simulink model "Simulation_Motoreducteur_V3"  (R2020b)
settings: Solver=FixedStepAuto  StartTime=0.0  StopTime=3  FixedStep=0.001  RelTol=1e-3
libraries: simulink x2

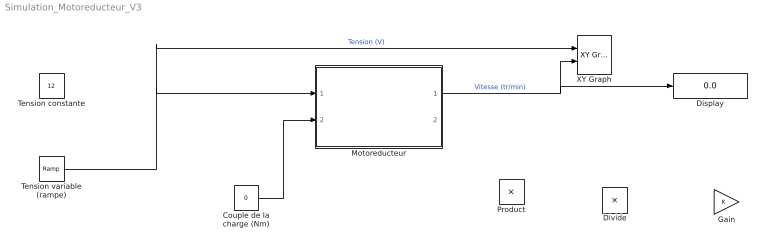
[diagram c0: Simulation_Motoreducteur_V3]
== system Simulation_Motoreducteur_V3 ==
  Couple de la charge (Nm) : Constant  Value=0
  Display : Display
  Divide : Product  Inputs=*/
  Gain : Gain
  Motoreducteur : Subsystem  mask{k=1, R=0, Io=0, r1=1, Rend=100}
      mask prompts: k "Constante de couple (Nm/A)"; R "Resistance d'induit (ohm)"; Io "Courant a vide (A)"; r1 "Rapport de reduction"; Rend "Rendement du reducteur (%)"
  Product : Product
  Tension constante : Constant  Value=12
  Tension variable (rampe) : simulink/Sources/Ramp  slope=12/3  start=0  InitialOutput=0
  XY Graph : simulink/Sinks/XY Graph  xmin=0  xmax=12  ymin=0  ymax=250  st=-1
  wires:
  Tension variable (rampe)/1 -> XY Graph/1, Motoreducteur/1(In1)  "Tension (V)"
  Motoreducteur/1(Out2) -> XY Graph/2, Display/1  "Vitesse (tr/min)"
  Motoreducteur/2(Out3) -> ?  "Courant (A)"
  Couple de la charge (Nm)/1 -> Motoreducteur/2(In2)

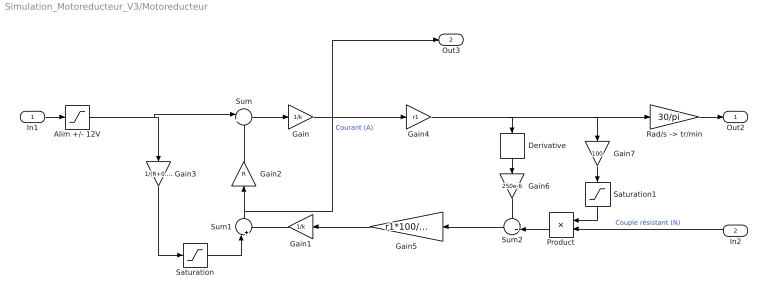
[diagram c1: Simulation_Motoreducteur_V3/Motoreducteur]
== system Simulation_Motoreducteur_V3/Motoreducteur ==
  In1 : Inport
  In2 : Inport  Port=2
  Alim +/- 12V : Saturate  UpperLimit=12  LowerLimit=-12
  Derivative : Derivative
  Gain : Gain  Gain=1/k
  Gain1 : Gain  Gain=1/k
  Gain2 : Gain  Gain=R
  Gain3 : Gain  Gain=1/(R+0.01)
  Gain4 : Gain  Gain=r1
  Gain5 : Gain  Gain=r1*100/Rend
  Gain6 : Gain  Gain=250e-6
  Gain7 : Gain  Gain=100
  Product : Product
  "Rad/s -> tr/min" : Gain  Gain=30/pi
  Saturation : Saturate  UpperLimit=Io  LowerLimit=-Io
  Saturation1 : Saturate  UpperLimit=1  LowerLimit=-1
  Sum : Sum  Inputs=|+-
  Sum1 : Sum  Inputs=|++
  Sum2 : Sum  Inputs=++|
  Out2 : Outport  VectorParamsAs1DForOutWhenUnconnected=off
  Out3 : Outport  Port=2  VectorParamsAs1DForOutWhenUnconnected=off
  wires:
  Alim +/- 12V/1 -> Sum/1, Gain3/1
  In1/1 -> Alim +/- 12V/1
  "Rad/s -> tr/min"/1 -> Out2/1
  Gain4/1 -> Derivative/1, Gain7/1, "Rad/s -> tr/min"/1
  Sum1/1 -> Out3/1, Gain2/1  "Courant (A)"
  Sum/1 -> Gain/1
  Gain2/1 -> Sum/2
  Gain3/1 -> Saturation/1
  Gain1/1 -> Sum1/2
  Saturation/1 -> Sum1/1
  Gain5/1 -> Gain1/1
  Gain/1 -> Gain4/1
  Gain6/1 -> Sum2/1
  Derivative/1 -> Gain6/1
  In2/1 -> Product/2  "Couple résistant (N)"
  Sum2/1 -> Gain5/1
  Product/1 -> Sum2/2
  Saturation1/1 -> Product/1
  Gain7/1 -> Saturation1/1
